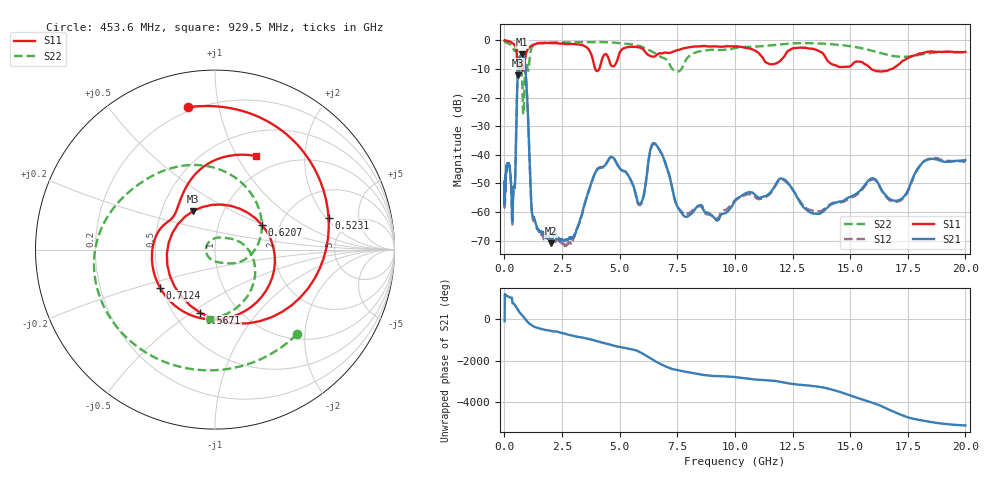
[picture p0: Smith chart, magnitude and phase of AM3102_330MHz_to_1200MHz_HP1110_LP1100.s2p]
! Date/Time: Tue, Sep 11, 2018 5:23 PM
! Network Analyzer: Agilent Technologies E8362B Rev: A.07.50.63
! Sweep from 0.010 to 20.000 GHz, 1601 Points, Sweep Type: LOG
! Power Supply: 4.949 V, 0.001 A
# Hz S DB R 50
!freq MagS11 AngS11 MagS21 AngS21 MagS12 AngS12 MagS22 AngS22
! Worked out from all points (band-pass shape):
!   1601 points, 10 MHz to 20 GHz, reference 50 ohm
!   highest |S21| = -4.86 dB at 768.6 MHz (marker M1); lowest = -71.0 dB at 2.035 GHz (marker M2)
!   |S21| within 3 dB of the highest: 609.2 MHz to 884 MHz (274.8 MHz wide, 36.8 % of centre)
!   lowest |S11| = -12.1 dB at 597.5 MHz (marker M3), VSWR 1.66, Z = 36.1 + j16.6 ohm
!   |S11| at or under -10 dB: 780.2 MHz to 838.2 MHz (58.01 MHz wide, 7.17 % of centre); 3.941 GHz to 4.114 GHz (172.8 MHz wide, 4.29 % of centre); 15.91 GHz to 16.81 GHz (897.2 MHz wide, 5.48 % of centre)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
!   |S22| runs from -25.9 to -0.3 dB; largest |S21 - S12| = 0.0082
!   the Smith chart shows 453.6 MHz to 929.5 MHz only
!   S11 on the Smith chart (normalised r, x): 453.6 MHz: 0.18, +0.81; 523.1 MHz: 3.42, +2.13; 567.1 MHz: 0.67, -0.54; 620.7 MHz: 1.61, +0.49; 712.4 MHz: 0.49, -0.24; 929.5 MHz: 0.78, +1.20
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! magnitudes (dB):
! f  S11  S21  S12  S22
! 10 MHz  0.0  -50.2  -49.2  -0.3
! 35.55 MHz  -0.1  -51.8  -51.6  -0.5
! 126.4 MHz  -0.2  -43.2  -43.3  -0.9
! 339.5 MHz  -1.0  -63.2  -64.2  -2.2
! 447.2 MHz  -1.8  -51.6  -51.5  -3.7
! 453.6 MHz  -1.9  -51.0  -51.1  -3.7
! 523.1 MHz  -3.6  -27.3  -27.4  -3.1
! 567.1 MHz  -8.8  -13.9  -13.8  -3.7
! 597.5 MHz  -12.1  -8.9  -9.0  -4.7
! 620.7 MHz  -10.6  -7.2  -7.4  -5.3
! 712.4 MHz  -8.6  -5.2  -5.2  -8.6
! 768.6 MHz  -9.7  -4.9  -4.9  -13.9
! 929.5 MHz  -4.9  -11.9  -12.0  -8.3
! 1.201 GHz  -1.7  -60.5  -60.9  -2.3
! 1.59 GHz  -1.0  -66.7  -67.7  -0.9
! 2.035 GHz  -1.0  -71.0  -69.2  -0.7
! 4.608 GHz  -8.5  -40.8  -40.7  -0.7
! 5.652 GHz  -2.3  -52.3  -52.6  -1.6
! 6.58 GHz  -5.3  -36.5  -36.6  -4.7
! 7.808 GHz  -2.7  -61.4  -60.8  -7.9
! 13.55 GHz  -3.4  -60.6  -59.8  -1.1
! 20 GHz  -4.1  -41.8  -42.4  -4.2
